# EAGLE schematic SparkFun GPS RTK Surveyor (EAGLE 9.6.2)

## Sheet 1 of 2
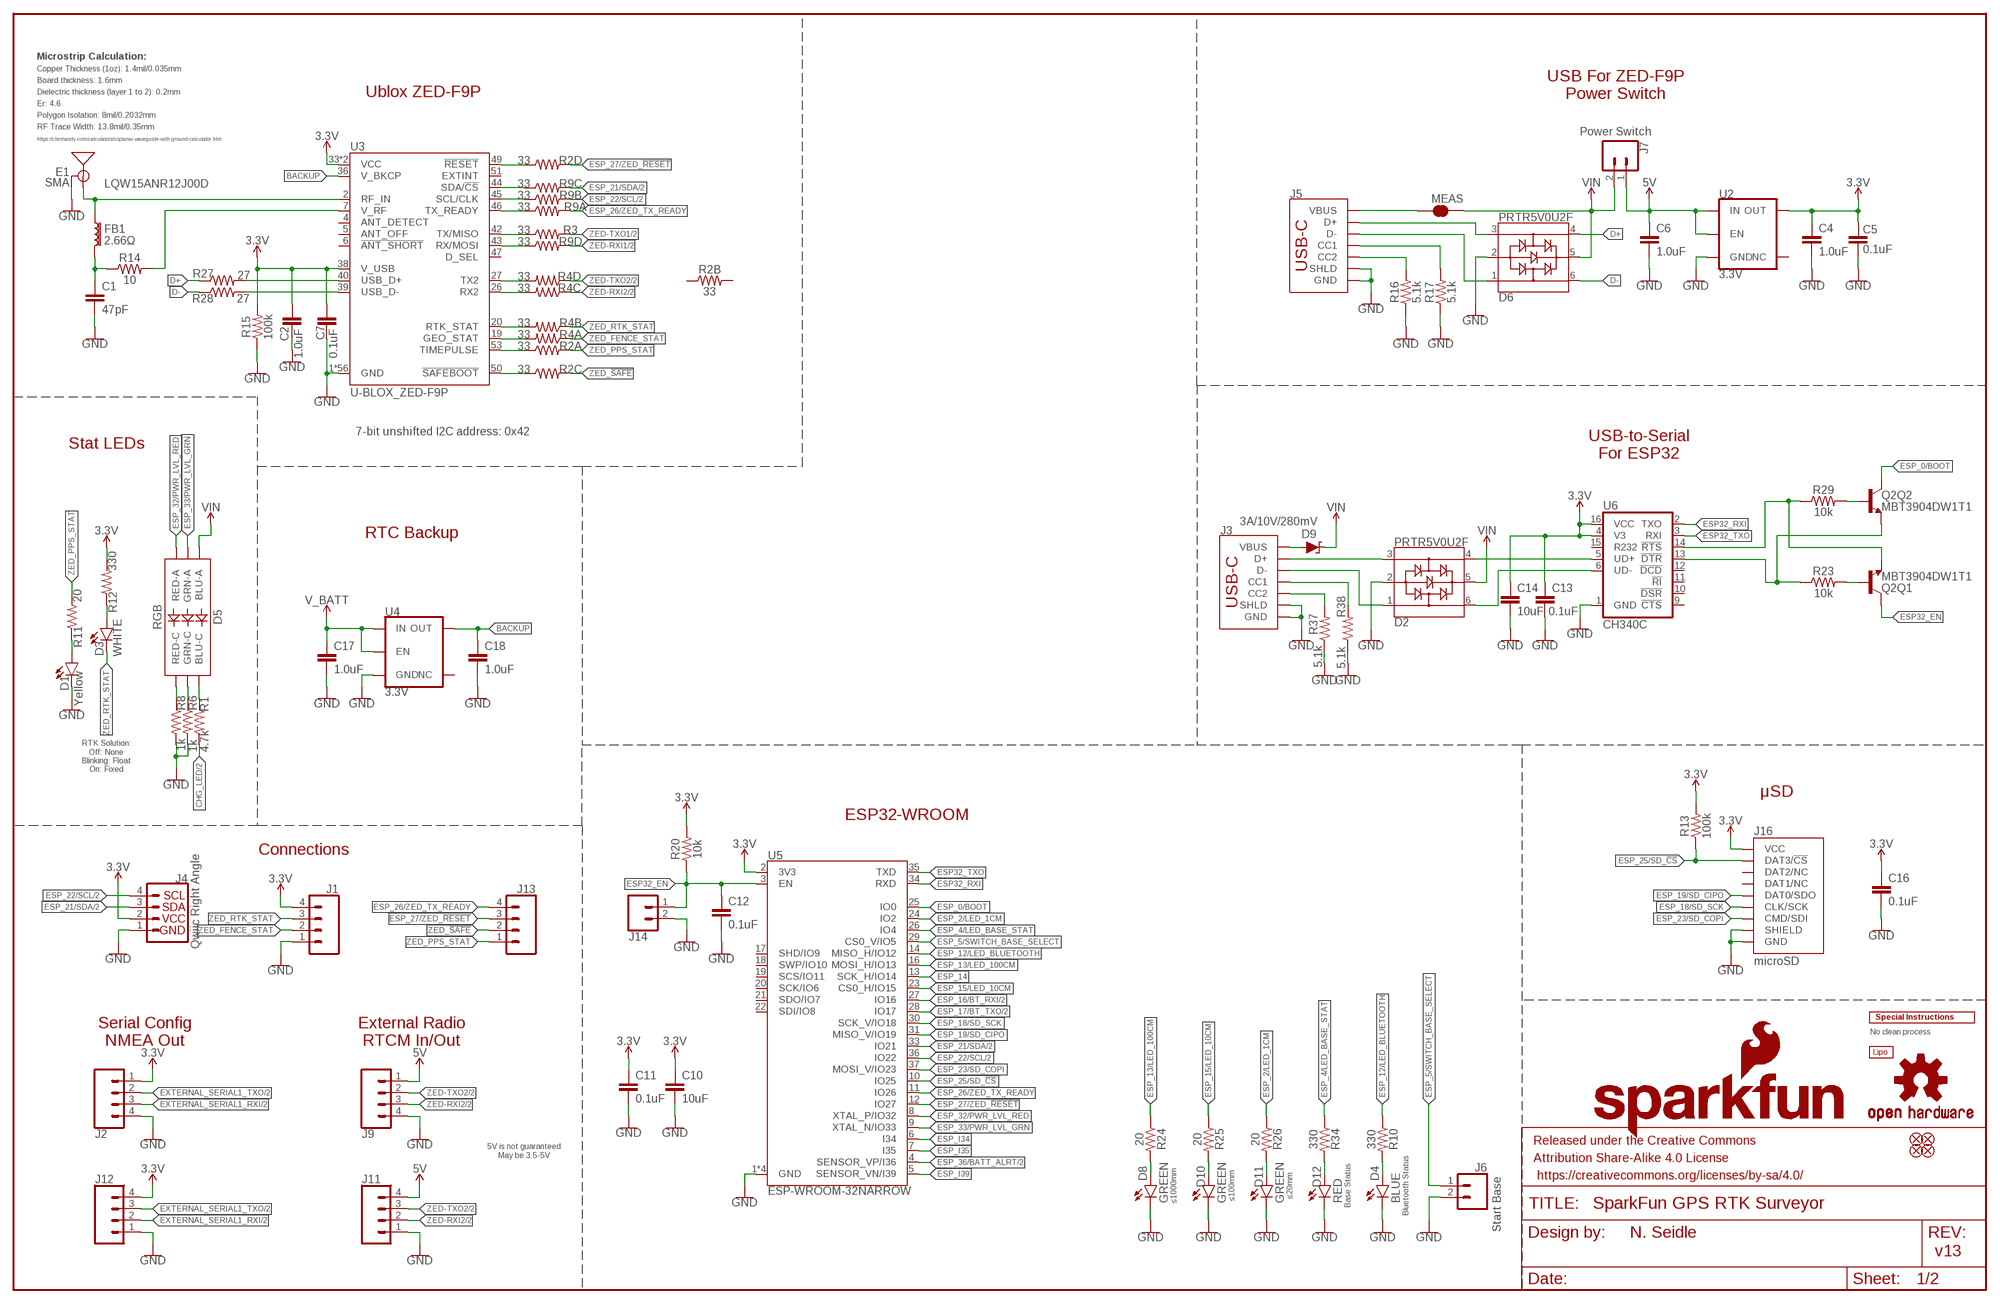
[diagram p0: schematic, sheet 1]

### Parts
BT1  LIPO-OUTLINE1100  [LIPO-1000]
C1  47pF  47PF-0402-25V-5%-X7R  [0402]
C2  1.0uF  1.0UF-0603-16V-10%-X7R  [0603]
C4  1.0uF  1.0UF-0603-16V-10%-X7R  [0603]
C5  0.1uF  0.1UF-0603-25V-5%  [0603]
C6  1.0uF  1.0UF-0603-16V-10%-X7R  [0603]
C7  0.1uF  0.1UF-0603-25V-5%  [0603]
C10  10uF  10UF-0603-6.3V-20%  [0603]
C11  0.1uF  0.1UF-0603-25V-(+80/-20%)  [0603]
C12  0.1uF  0.1UF-0603-25V-(+80/-20%)  [0603]
C13  0.1uF  0.1UF-0603-25V-(+80/-20%)  [0603]
C14  10uF  10UF-0603-6.3V-20%  [0603]
C16  0.1uF  0.1UF-0603-25V-(+80/-20%)  [0603]
C17  1.0uF  1.0UF-0603-16V-10%-X7R  [0603]
C18  1.0uF  1.0UF-0603-16V-10%-X7R  [0603]
D1  Yellow  LED-YELLOW0603  [LED-0603]
D2  PRTR5V0U2F  [SOT886]
D3  WHITE  LED-WHITE0603  [LED-0603]
D4  BLUE  LED-BLUE0603  [LED-0603]
D5  RGB  LED-RGBPLCC-6  [PLCC-6-LED]
D6  PRTR5V0U2F  [SOT886]
D8  GREEN  LED-GREEN0603  [LED-0603]
D9  3A/10V/280mV  DIODE-SCHOTTKY-BAT60A  [SOD-323]
D10  GREEN  LED-GREEN0603  [LED-0603]
D11  GREEN  LED-GREEN0603  [LED-0603]
D12  RED  LED-RED0603  [LED-0603]
E1  SMA  ANTENNA-SMA-GROUNDEDEDGE_SMA_SMD  [SMA-EDGE-SMD]
FB1  2.66Ω  FERRITE_BEAD-0402-2.66OHM-1GHZ  [0402-TIGHT]
FRAME2  FRAME-LEDGER  [CREATIVE_COMMONS]
J1  CONN_041X04_NO_SILK_NO_POP  [1X04_NO_SILK]
J2  CONN_04JST-SMD-LOCKING  [JST-4-SMD-1.25MM-LOCKING]
J3  USB Female Type C Connector  USB_C_4-LAYER_PADS  [USB-C-16P_4LAYER-PADS]
J4  Qwiic Right Angle  I2C_STANDARDQWIIC  [JST04_1MM_RA]
J5  USB Female Type C Connector  USB_C_4-LAYER_PADS  [USB-C-16P_4LAYER-PADS]
J6  Start Base  CONN_02-JST-2MM-SMT  [JST-2-SMD]
J7  Power Switch  CONN_02-JST-2MM-SMT  [JST-2-SMD]
J9  CONN_04JST-SMD-LOCKING  [JST-4-SMD-1.25MM-LOCKING]
J11  CONN_041X04_NO_SILK_NO_POP  [1X04_NO_SILK]
J12  CONN_041X04_NO_SILK_NO_POP  [1X04_NO_SILK]
J13  CONN_041X04_NO_SILK_NO_POP  [1X04_NO_SILK]
J14  CONN_021X02_NO_SILK  [1X02_NO_SILK]
J16  microSD  MICRO-SD-SDIOPUSH-PUSH  [MICRO-SD-SOCKET]
JP21  FIDUCIALUFIDUCIAL  [FIDUCIAL-MICRO]
JP61  FIDUCIALUFIDUCIAL  [FIDUCIAL-MICRO]
JP71  FIDUCIALUFIDUCIAL  [FIDUCIAL-MICRO]
JP81  FIDUCIALUFIDUCIAL  [FIDUCIAL-MICRO]
LOGO1  OSHW-LOGOMINI  [OSHW-LOGO-MINI]
LOGO2  SFE_LOGO_NAME_FLAME.1_INCH  [SFE_LOGO_NAME_FLAME_.1]
MEAS  JUMPER-COMBO_2_NC_TRACE  [COMBO-JUMPER_2_NC_TRACE]
Q2  MBT3904DW1T1  TRANS_NPN_DUAL-MBT3904DW1T1  [SC70-6]
R1  4.7k  4.7KOHM-0603-1/10W-1%  [0603]
R2  33  33OHM_RA-1206-1/16W-5%  [1206_RA]
R3  33  33OHM-0603-1/10W-1%  [0603]
R4  33  33OHM_RA-1206-1/16W-5%  [1206_RA]
R6  1k  1KOHM-0603-1/10W-1%  [0603]
R8  1k  1KOHM-0603-1/10W-1%  [0603]
R9  33  33OHM_RA-1206-1/16W-5%  [1206_RA]
R10  330  330OHM-0603-1/10W-1%  [0603]
R11  20  20OHM-0603-1/10W-1%  [0603]
R12  330  330OHM-0603-1/10W-1%  [0603]
R13  100k  100KOHM-0603-1/10W-1%  [0603]
R14  10  10OHM-0603-1/10W-1%  [0603]
R15  100k  100KOHM-0603-1/10W-1%  [0603]
R16  5.1k  5.1KOHM5.1KOHM-0603-1/10W-1%  [0603]
R17  5.1k  5.1KOHM5.1KOHM-0603-1/10W-1%  [0603]
R20  10k  10KOHM-0603-1/10W-1%  [0603]
R23  10k  10KOHM-0603-1/10W-1%  [0603]
R24  20  20OHM-0603-1/10W-1%  [0603]
R25  20  20OHM-0603-1/10W-1%  [0603]
R26  20  20OHM-0603-1/10W-1%  [0603]
R27  27  27OHM-0603-1/10W-1%  [0603]
R28  27  27OHM-0603-1/10W-1%  [0603]
R29  10k  10KOHM-0603-1/10W-1%  [0603]
R34  330  330OHM-0603-1/10W-1%  [0603]
R37  5.1k  5.1KOHM5.1KOHM-0603-1/10W-1%  [0603]
R38  5.1k  5.1KOHM5.1KOHM-0603-1/10W-1%  [0603]
U2  3.3V  V_REG_AP2112K-3.3V  [SOT23-5]
U3  U-BLOX_ZED-F9P  [ZED-F9P]
U4  3.3V  V_REG_AP2112K-3.3V  [SOT23-5]
U5  ESP-WROOM-32NARROW  [ESP-WROOM-32-NARROW]
U6  CH340C  [SO016]
U$2  SPECIAL_INSTRUCTIONS-ORDERING  [ORDERING_INSTRUCTIONS]

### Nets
3.3V [power]: C2.1 C4.1 C5.2 C7.2 C10.1 C11.1 C13.1 C14.1 C16.1 J1.4 J2.1 J4.2 J12.4 J16.VCC R12.2 R13.2 R15.2 R20.2 U2.5(OUT) U3.33(VCC) U3.34(VCC) U3.38(V_USB) U5.2(3V3) U6.4(V3) U6.16(VCC)
5V [power]: C6.1 J7.1 J9.1 J11.4 U2.1(IN) U2.3(EN)
ANT_VCC: C1.1 FB1.2 R14.1
BACKUP: C18.1 U3.36(V_BKCP) U4.5(OUT)
CC1: J5.A5(CC1) R17.2
CC2: J5.B5(CC2) R16.2
CC3: J3.B5(CC2) R37.2
CC4: J3.A5(CC1) R38.2
CHG_LED: R1.2 ; also sheet 2
D+: D6.4 R27.1
D+1: D2.4 U6.5(UD+)
D-: D6.6 R28.1
D-1: D2.6 U6.6(UD-)
ESP32_!DTR: Q2.1(Q2:E) R23.1 U6.13(!DTR)
ESP32_!RTS: Q2.4(Q1:E) R29.1 U6.14(!RTS)
ESP32_EN: C12.1 J14.1 Q2.3(Q1:C) R20.1 U5.3(EN)
ESP32_RXI: U5.34(RXD) U6.2(TXO)
ESP32_TXO: U5.35(TXD) U6.3(RXI)
ESP_0/BOOT: Q2.6(Q2:C) U5.25(IO0)
ESP_2/LED_1CM: R26.1 U5.24(IO2)
ESP_4/LED_BASE_STAT: R34.1 U5.26(IO4)
ESP_5/SWITCH_BASE_SELECT: J6.1 U5.29(CS0_V/IO5)
ESP_12/LED_BLUETOOTH: R10.1 U5.14(MISO_H/IO12)
ESP_13/LED_100CM: R24.1 U5.16(MOSI_H/IO13)
ESP_14: U5.13(SCK_H/IO14)
ESP_15/LED_10CM: R25.1 U5.23(CS0_H/IO15)
ESP_16/BT_RXI: U5.27(IO16) ; also sheet 2
ESP_17/BT_TXO: U5.28(IO17) ; also sheet 2
ESP_18/SD_SCK: J16.SCLK(CLK/SCK) U5.30(SCK_V/IO18)
ESP_19/SD_CIPO: J16.DO/DAT0(DAT0/SDO) U5.31(MISO_V/IO19)
ESP_21/SDA: J4.3 R9.P6 U5.33(IO21) ; also sheet 2
ESP_22/SCL: J4.4 R9.P7 U5.36(IO22) ; also sheet 2
ESP_23/SD_COPI: J16.DI/CMD(CMD/SDI) U5.37(MOSI_V/IO23)
ESP_25/SD_!CS!: J16.CS/DAT3(DAT3/!CS!) R13.1 U5.10(IO25)
ESP_26/ZED_TX_READY: J13.4 R9.P8 U5.11(IO26)
ESP_27/ZED_!RESET!: J13.3 R2.P5 U5.12(IO27)
ESP_32/PWR_LVL_RED: D5.AR(RED-A) U5.8(XTAL_P/IO32)
ESP_33/PWR_LVL_GRN: D5.AG(GRN-A) U5.9(XTAL_N/IO33)
ESP_36/BATT_ALRT: U5.4(SENSOR_VP/I36) ; also sheet 2
ESP_D1+: D2.3 J3.A6(D+) J3.B6(D+)
ESP_D1-: D2.1 J3.A7(D-) J3.B7(D-)
ESP_I34: U5.6(I34)
ESP_I35: U5.7(I35)
ESP_I39: U5.5(SENSOR_VN/I39)
EXTERNAL_SERIAL1_RXI: J2.3 J12.2 ; also sheet 2
EXTERNAL_SERIAL1_TXO: J2.2 J12.3 ; also sheet 2
FENCE_LV: R4.P8 U3.19(GEO_STAT)
GND: C1.2 C2.2 C4.2 C5.1 C6.2 C7.1 C10.2 C11.2 C12.2 C13.2 C14.2 C16.2 C17.2 C18.2 D1.C D2.2 D4.C D6.2 D8.C D10.C D11.C D12.C E1.GND@0(GND) E1.GND@1(GND) J1.1 J2.4 J3.GND J3.GND2(GND) J3.SHLD1(SHLD) J3.SHLD2(SHLD) J3.SHLD3(SHLD) J3.SHLD4(SHLD) J4.1 J5.GND J5.GND2(GND) J5.SHLD1(SHLD) J5.SHLD2(SHLD) J5.SHLD3(SHLD) J5.SHLD4(SHLD) J6.2 J9.4 J11.1 J12.1 J14.2 J16.CD1(SHIELD) J16.GND J16.GND1(GND) J16.GND3(GND) R6.2 R8.2 R15.1 R16.1 R17.1 R37.1 R38.1 U2.2(GND) U3.1(GND) U3.3(GND) U3.12(GND) U3.14(GND) U3.32(GND) U3.37(GND) U3.41(GND) U3.48(GND) U3.55(GND) U3.56(GND) U3.57(GND) U3.58(GND) U3.59(GND) U3.60(GND) U3.61(GND) U3.62(GND) U3.63(GND) U3.64(GND) U3.65(GND) U3.66(GND) U3.67(GND) U3.68(GND) U3.69(GND) U3.70(GND) U3.71(GND) U3.72(GND) U3.73(GND) U3.74(GND) U3.75(GND) U3.76(GND) U3.77(GND) U3.78(GND) U3.79(GND) U3.80(GND) U3.81(GND) U3.82(GND) U3.83(GND) U3.84(GND) U3.85(GND) U3.86(GND) U3.87(GND) U3.88(GND) U3.89(GND) U3.90(GND) U3.91(GND) U3.92(GND) U3.93(GND) U3.94(GND) U3.95(GND) U3.96(GND) U3.97(GND) U3.98(GND) U3.99(GND) U3.100(GND) U3.101(GND) U3.102(GND) U4.2(GND) U5.1(GND) U5.15(GND) U5.38(GND) U5.GND U6.1(GND) ; also sheet 2
GPS_ANT1 [RF]: E1.SIG(SIGNAL) FB1.1 U3.2(RF_IN)
N$1: D3.A R12.1
N$2: D1.A R11.1
N$3: D4.A R10.2
N$4 [power]: J5.VBUS1(VBUS) J5.VBUS2(VBUS) MEAS.1 MEAS.3
N$10: D5.CG(GRN-C) R6.1
N$11: R27.2 U3.40(USB_D+)
N$12: R28.2 U3.39(USB_D-)
N$13: R14.2 U3.7(V_RF)
N$14: D5.CR(RED-C) R8.1
N$16: R2.P4 U3.49(!RESET!)
N$17: D5.CB(BLU-C) R1.1
N$18: R2.P3 U3.50(!SAFEBOOT!)
N$22: R9.P1 U3.46(TX_READY)
N$24: Q2.5(Q1:B) R23.2
N$25: Q2.2(Q2:B) R29.2
N$26: D8.A R24.2
N$27: D10.A R25.2
N$29: D11.A R26.2
N$30: D12.A R34.2
N$32 [power]: D9.A J3.VBUS1(VBUS) J3.VBUS2(VBUS)
PPS: R2.P1 U3.53(TIMEPULSE)
RTK_LV: R4.P7 U3.20(RTK_STAT)
RX2_LV: R4.P6 U3.26(RX2)
RXLV: R9.P4 U3.43(RX/MOSI)
SCL_LV: R9.P2 U3.45(SCL/CLK)
SDA_LV: R9.P3 U3.44(SDA/!CS!)
TX2_LV: R4.P5 U3.27(TX2)
TXLV: R3.1 U3.42(TX/MISO)
UNP_D+: D6.3 J5.A6(D+) J5.B6(D+)
UNP_D-: D6.1 J5.A7(D-) J5.B7(D-)
V_BATT [power]: C17.1 U4.1(IN) U4.3(EN) ; also sheet 2
VIN [power]: D2.5 D5.AB(BLU-A) D6.5 D9.C J7.2 MEAS.2 MEAS.4 ; also sheet 2
ZED-RXI1: R9.P5 ; also sheet 2
ZED-RXI2: J9.3 J11.2 R4.P3 ; also sheet 2
ZED-TXO1: R3.2 ; also sheet 2
ZED-TXO2: J9.2 J11.3 R4.P4 ; also sheet 2
ZED_!SAFE!: J13.2 R2.P6
ZED_FENCE_STAT: J1.2 R4.P1
ZED_PPS_STAT: J13.1 R2.P8 R11.2
ZED_RTK_STAT: D3.C J1.3 R4.P2
Unconnected: J16.DAT1(DAT1/NC) J16.DAT2(DAT2/NC) R2.P2 R2.P7 U2.4(NC) U3.4(ANT_DETECT) U3.5(ANT_OFF) U3.6(!ANT_SHORT!) U3.47(D_SEL) U3.51(EXTINT) U4.4(NC) U5.17(SHD/IO9) U5.18(SWP/IO10) U5.19(SCS/IO11) U5.20(SCK/IO6) U5.21(SDO/IO7) U5.22(SDI/IO8) U6.9(!CTS) U6.10(!DSR) U6.11(!RI) U6.12(!DCD) U6.15(R232)

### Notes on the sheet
- Microstrip Calculation:
- Copper Thickness (1oz): 1.4mil/0.035mm
- Board thickness: 1.6mm
- USB For ZED-F9P
  Power Switch
- Ublox ZED-F9P
- Dielectric thickness (layer 1 to 2): 0.2mm
- Er: 4.6
- Polygon Isolation: 8mil/0.2032mm
- RF Trace Width: 13.8mil/0.35mm
- https://chemandy.com/calculators/coplanar-waveguide-with-ground-calculator.htm
- LQW15ANR12J00D
- 7-bit unshifted I2C address: 0x42
- Stat LEDs
- USB-to-Serial
  For ESP32
- RTC Backup
- RTK Solution:
  Off: None
  Blinking: Float
  On: Fixed
- μSD
- ESP32-WROOM
- Connections
- Serial Config
  NMEA Out
- External Radio
  RTCM In/Out
- No clean process
- 5V is not guaranteed
  May be 3.5-5V
- ≤1000mm | ≤100mm | ≤20mm | Base Status | Bluetooth Status
- N. Seidle
- v13

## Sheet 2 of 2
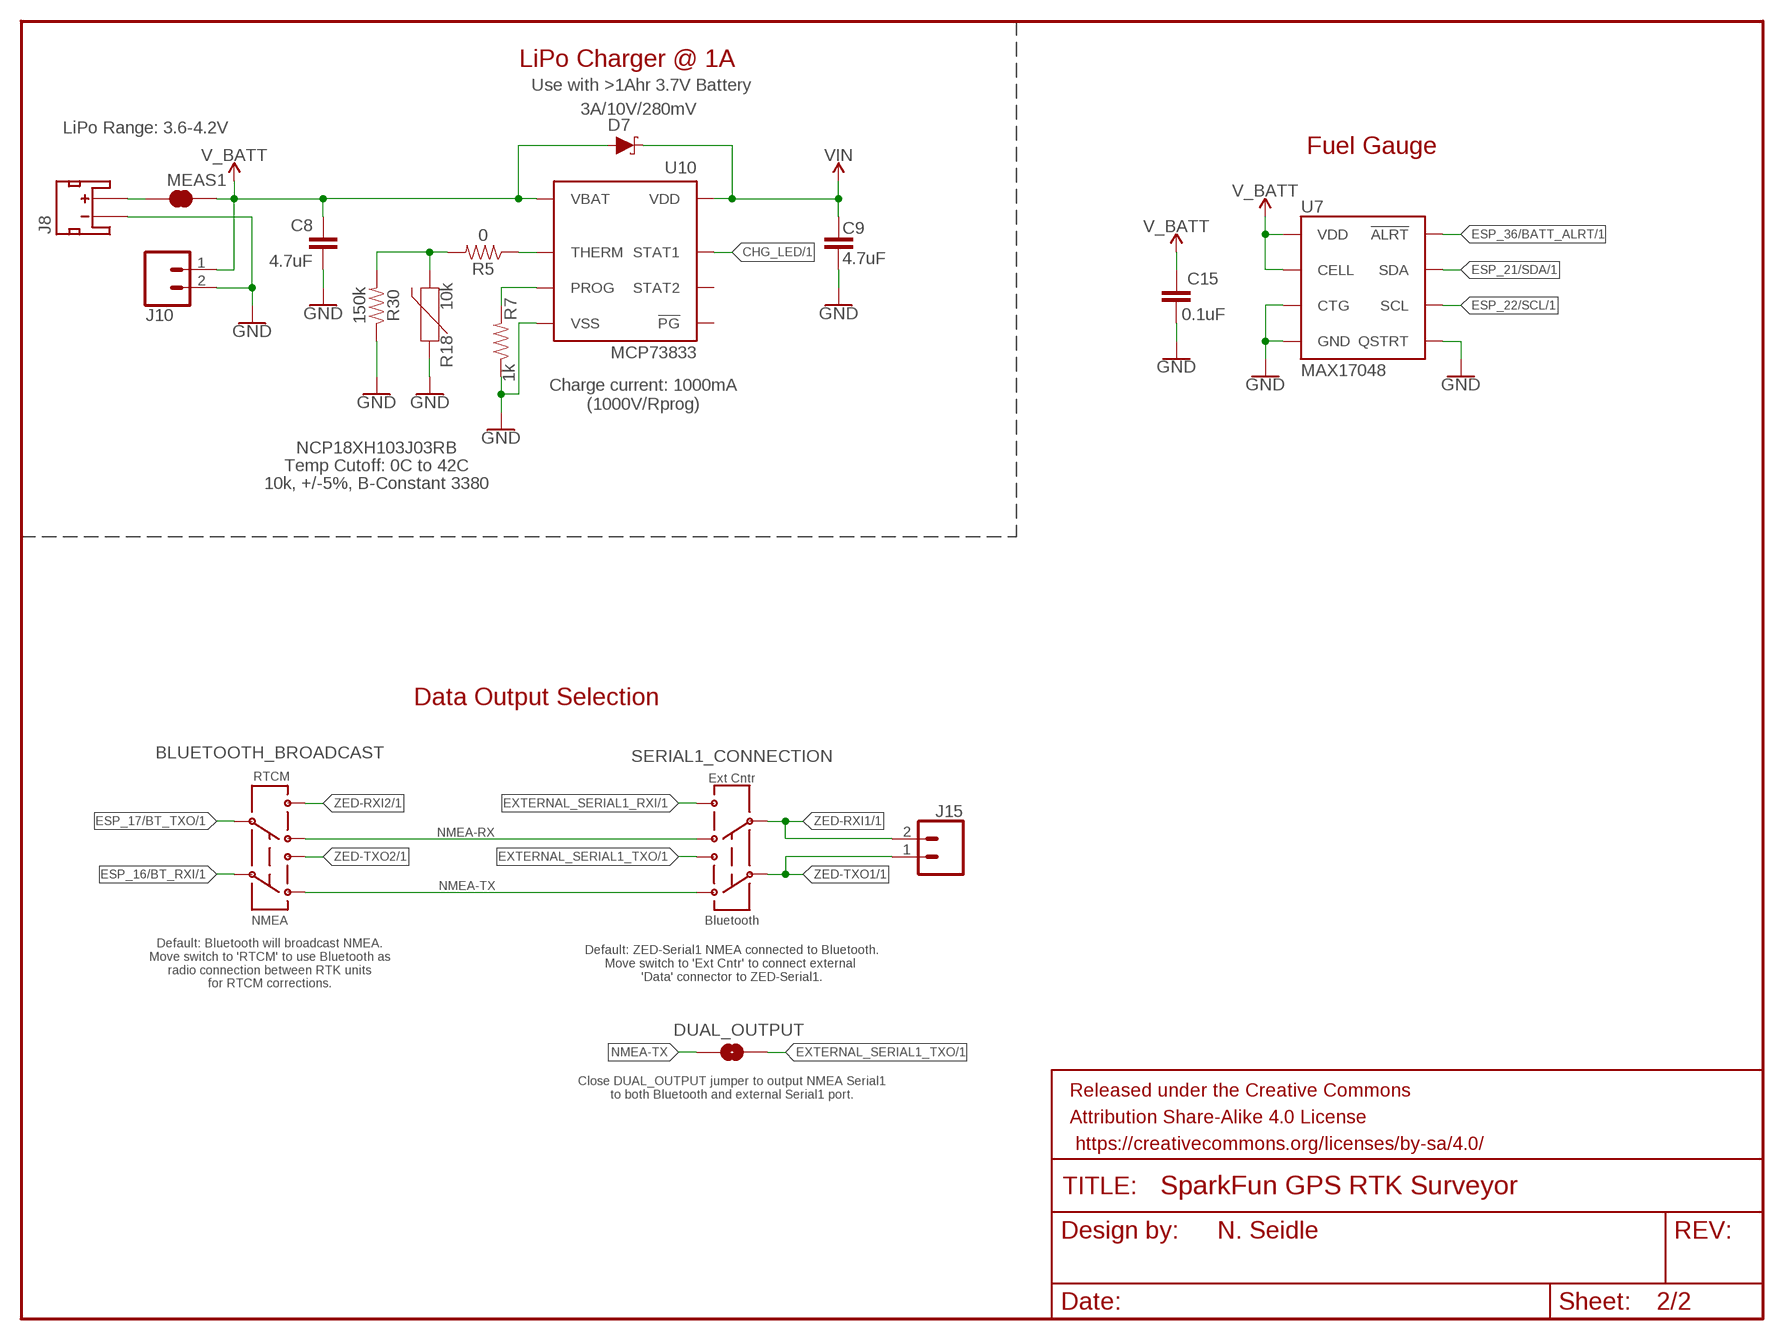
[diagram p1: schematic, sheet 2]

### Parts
BLUETOOTH_BROADCAST  SWITCH-DPDT-SMD-AYZ0202  [SWITCH_DPDT_SMD_AYZ0202]
C8  4.7uF  4.7UF-0603-35V-(20%)  [0603]
C9  4.7uF  4.7UF-0603-35V-(20%)  [0603]
C15  0.1uF  0.1UF-0603-25V-(+80/-20%)  [0603]
D7  3A/10V/280mV  DIODE-SCHOTTKY-BAT60A  [SOD-323]
DUAL_OUTPUT  JUMPER-SMT_2_NO_SILK  [SMT-JUMPER_2_NO_SILK]
FRAME1  FRAME-LETTERNO_PACKAGE  [DUMMY]
J8  JST_2MM_MALE  [JST-2-SMD]
J10  CONN_021X02_NO_SILK  [1X02_NO_SILK]
J15  CONN_021X02_NO_SILK  [1X02_NO_SILK]
MEAS1  JUMPER-COMBO_2_NC_TRACE  [COMBO-JUMPER_2_NC_TRACE]
R5  0  0OHM-0603-1/10W  [0603]
R7  1k  1KOHM-0603-1/10W-1%  [0603]
R18  10k  NTC-THERMISTOR-0603  [0603]
R30  150k  150KOHM-0603-1/10W-1%  [0603]
SERIAL1_CONNECTION  SWITCH-DPDT-SMD-AYZ0202  [SWITCH_DPDT_SMD_AYZ0202]
U7  MAX17048  MAX17048DFN8  [DFN-8]
U10  MCP73833  [DFN-10]

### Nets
CHG_LED: U10.3(STAT1) ; also sheet 1
CHG_THERM1: R5.2 R18.2 R30.2
ESP_16/BT_RXI: BLUETOOTH_BROADCAST.2 ; also sheet 1
ESP_17/BT_TXO: BLUETOOTH_BROADCAST.5 ; also sheet 1
ESP_21/SDA: U7.8(SDA) ; also sheet 1
ESP_22/SCL: U7.7(SCL) ; also sheet 1
ESP_36/BATT_ALRT: U7.5(!ALRT) ; also sheet 1
EXTERNAL_SERIAL1_RXI: SERIAL1_CONNECTION.4 ; also sheet 1
EXTERNAL_SERIAL1_TXO: DUAL_OUTPUT.2 SERIAL1_CONNECTION.1 ; also sheet 1
GND: C8.2 C9.2 C15.2 J8.1(-) J10.2 R7.1 R18.1 R30.1 U7.1(CTG) U7.4(GND) U7.6(QSTRT) U7.9(GND) U10.5(VSS) U10.11(VSS) ; also sheet 1
LIPO_RAW: J8.2(+) MEAS1.1 MEAS1.3
N$5: R5.1 U10.8(THERM)
NMEA-RX: BLUETOOTH_BROADCAST.6 SERIAL1_CONNECTION.6
NMEA-TX: BLUETOOTH_BROADCAST.3 DUAL_OUTPUT.1 SERIAL1_CONNECTION.3
PROG1: R7.2 U10.6(PROG)
V_BATT [power]: C8.1 C15.1 D7.A J10.1 MEAS1.2 MEAS1.4 U7.2(CELL) U7.3(VDD) U10.9(VBAT) U10.10(VBAT) ; also sheet 1
VIN [power]: C9.1 D7.C U10.1(VDD) U10.2(VDD) ; also sheet 1
ZED-RXI1: J15.2 SERIAL1_CONNECTION.5 ; also sheet 1
ZED-RXI2: BLUETOOTH_BROADCAST.4 ; also sheet 1
ZED-TXO1: J15.1 SERIAL1_CONNECTION.2 ; also sheet 1
ZED-TXO2: BLUETOOTH_BROADCAST.1 ; also sheet 1
Unconnected: J8.NC1(PAD1) J8.NC2(PAD2) U10.4(STAT2) U10.7(!PG)

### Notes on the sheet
- LiPo Charger @ 1A
- Use with >1Ahr 3.7V Battery
- LiPo Range: 3.6-4.2V
- Fuel Gauge
- Charge current: 1000mA
  (1000V/Rprog)
- NCP18XH103J03RB
- Temp Cutoff: 0C to 42C
- 10k, +/-5%, B-Constant 3380
- Data Output Selection
- RTCM | Ext Cntr
- NMEA | Bluetooth
- Default: Bluetooth will broadcast NMEA.
  Move switch to 'RTCM' to use Bluetooth as
  radio connection between RTK units
  for RTCM corrections.
- Default: ZED-Serial1 NMEA connected to Bluetooth.
  Move switch to 'Ext Cntr' to connect external 
  'Data' connector to ZED-Serial1.
- Close DUAL_OUTPUT jumper to output NMEA Serial1
  to both Bluetooth and external Serial1 port.
- N. Seidle

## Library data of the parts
BLUETOOTH_BROADCAST SERIAL1_CONNECTION = SparkFun-Switches:SWITCH-DPDT: Double-Pole, Double-Throw (DPDT) Switch Double-pole, double-throw switches. Variant Overview PTH-GPI-152-3013 Used on SparkFun Geiger Counter SMD-AY0202 Surface Mount DPDT Switch (COM-00597) Used on e.g. LilyPad Arduino USB - ATmega32U4 Board; PROD_ID: SWCH-08179; SF_SKU: COM-00597
BT1 = SparkFun-Batteries:LIPO-OUTLINE: LiPo Battery Outlines; PROD_ID: BATT-13243; SF_SKU: PRT-13813
C1 = SparkFun-Capacitors:47PF: 47pF ceramic capacitors; PROD_ID: CAP-15063
C2 C4 C6 C17 C18 = SparkFun-Capacitors:1.0UF: 1µF ceramic capacitors; PROD_ID: CAP-13930
C5 C7 = SparkFun-Capacitors:0.1UF: 0.1µF ceramic capacitors; PROD_ID: CAP-08604
C8 C9 = SparkFun-Capacitors:4.7UF: 4.7µF ceramic capacitors; PROD_ID: CAP-14106
C10 C14 = SparkFun-Capacitors:10UF: 10.0µF ceramic capacitors; PROD_ID: CAP-11015
C11-C13 C15 C16 = SparkFun-Capacitors:0.1UF: 0.1µF ceramic capacitors; PROD_ID: CAP-00810
D1 = SparkFun-LED:LED-YELLOW: Yellow SMD LED; PROD_ID: DIO-09003
D2 D6 = SparkFun-IC-Power:PRTR5V0U2: A small ESD protection device. Most commonly used on USB D+/D- signals to protect large, expensive, or especially sensitive USB enabled devices.; PROD_ID: DIO-14084
D3 = SparkFun-LED:LED-WHITE: White SMD LED; PROD_ID: DIO-09004
D4 = SparkFun-LED:LED-BLUE: Blue SMD LED; PROD_ID: DIO-08575
D5 = SparkFun-LED:LED-RGB: LED-RGB 6 pin RGB LED (no common connector) Packages: PLCC-6 LED-TRICOLOR-5050 - No built-in IC SparkFun Products: Digital Sandbox LED- SMD RGB; PROD_ID: DIO-12113
D7 D9 = SparkFun-DiscreteSemi:DIODE-SCHOTTKY: Schottky diode; PROD_ID: DIO-14072
D8 D10 D11 = SparkFun-LED:LED-GREEN: Green SMD LED; PROD_ID: DIO-00821
D12 = SparkFun-LED:LED-RED: Red SMD LED; PROD_ID: DIO-00819
DUAL_OUTPUT = SparkFun-Jumpers:JUMPER-SMT_2_NO: Normally open jumper
E1 = SparkFun-RF:ANTENNA-SMA-GROUNDED: SMA Antenna Connector w/ Ground; PROD_ID: CONN-15100
FB1 = SparkFun-Coils:FERRITE_BEAD: Ferrite Bead (blocks, cores, rings, chokes, etc.); PROD_ID: NDUC-15072
FRAME1 = SparkFun-Aesthetics:FRAME-LETTER: Schematic Frame - Letter; DESIGNER: Nobody; VERSION: v01
FRAME2 = SparkFun-Aesthetics:FRAME-LEDGER: Schematic Frame - Ledger
J1 J11-J13 = SparkFun-Connectors:CONN_04: Multi connection point. Often used as Generic Header-pin footprint for 0.1 inch spaced/style header connections On any of the 0.1 inch spaced packages, you can populate with these: Break Away Headers - Straight (PRT-00116) Break Away Male Headers - Right Angle (PRT-00553) Female Headers (PRT-00115)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
J2 J9 = SparkFun-Connectors:CONN_04: Multi connection point. Often used as Generic Header-pin footprint for 0.1 inch spaced/style header connections On any of the 0.1 inch spaced packages, you can populate with these: Break Away Headers - Straight (PRT-00116) Break Away Male Headers - Right Angle (PRT-00553) Female Headers (PRT-00115)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; PROD_ID: CONN-15303
J3 J5 = SparkFun-Connectors:USB_C: USB Type C 16Pin Connector Super Speed pins not available on the 16-pin purely SMD connector so this part is best for USB 2.0 implementations. D1 and D2 are tied together enabling D+/- no matter which way the cable is plugged into the connector. The two channel configuration pins (CC1/2) are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; PROD_ID: CONN-14122
J4 = SparkFun-Connectors:I2C_STANDARD: SparkFun I2C Standard Pinout Header SparkFun has standardized on a pinout for all I2C based sensor breakouts. This pinout allows I2C boards to be plugged directly into the headers on Arduino Uno compatible boards, and to be daisy chained easily. Example SparkFun Products: SparkFun Atmospheric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; PROD_ID: CONN-13694
J6 J7 = SparkFun-Connectors:CONN_02: Multi connection point. Often used as Generic Header-pin footprint for 0.1 inch spaced/style header connections; PROD_ID: CONN-11443
J8 = SparkFun-Connectors:JST_2MM_MALE: JST 2MM MALE RA CONNECTOR Two pin, compact surface mount connector. Commonly used as a battery input connection point. We really like the solid locking feeling and high current rating on these small connectors. We use these all the time as battery connectors. Mates to single-cell LiPo batteries.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; PROD_ID: CONN-11443; SF_ID: PRT-08612
J10 J14 J15 = SparkFun-Connectors:CONN_02: Multi connection point. Often used as Generic Header-pin footprint for 0.1 inch spaced/style header connections
J16 = SparkFun-Connectors:MICRO-SD-SDIO: microSD Socket for Transflash Push-push type µSD socket. tDoc lines correctly indicate media card edge positions when inserting (unlocked, locked, depressed). NOTE: CD1 and CD2 are connected internally, and the default detect state of the socket is detect pin to ground. SparkFun Products: WAV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; PROD_ID: CONN-07820
JP21 JP61 JP71 JP81 = SparkFun-Aesthetics:FIDUCIAL: Fiducial Alignment Points
LOGO1 = SparkFun-Aesthetics:OSHW-LOGO: Open-Source Hardware (OSHW) Logo
LOGO2 = SparkFun-Aesthetics:SFE_LOGO_NAME_FLAME: SparkFun Font Logo w/ Flame
MEAS MEAS1 = SparkFun-Jumpers:JUMPER-COMBO_2_NC_TRACE
Q2 = SparkFun-DiscreteSemi:TRANS_NPN_DUAL: Dual NPN Transistors in Single Package The MBT3904W1 puts two general purpose 3904 NPN transistors in a single package. Datasheet SparkFun Products: SparkFun ESP32 Thing; PROD_ID: TRANS-13337
R1 = SparkFun-Resistors:4.7KOHM: 4.7kΩ resistor; PROD_ID: RES-07857
R2 R4 R9 = SparkFun-Resistors:33OHM_RA: EXB-38V330JV Four Resistory Array - AEC-Q200 Certified; PROD_ID: RES-15081
R3 = SparkFun-Resistors:33OHM: 33Ω resistor; PROD_ID: RES-08270
R5 = SparkFun-Resistors:0OHM: 0Ω resistor; PROD_ID: RES-08609
R6-R8 = SparkFun-Resistors:1KOHM: 1kΩ resistor; PROD_ID: RES-07856
R10 R12 R34 = SparkFun-Resistors:330OHM: 330Ω resistor; PROD_ID: RES-00818
R11 R24-R26 = SparkFun-Resistors:20OHM: RES-07862; PROD_ID: RES-07862
R13 R15 = SparkFun-Resistors:100KOHM: 100kΩ resistor; PROD_ID: RES-07828
R14 = SparkFun-Resistors:10OHM: 10Ω resistor; PROD_ID: RES-12581
R16 R17 R37 R38 = SparkFun-Resistors:5.1KOHM; PROD_ID: RES-12083
R18 = SparkFun-Resistors:NTC-THERMISTOR: NTC Thermistor; PROD_ID: RES-13608
R20 R23 R29 = SparkFun-Resistors:10KOHM: 10kΩ resistor; PROD_ID: RES-00824
R27 R28 = SparkFun-Resistors:27OHM: 27Ω resistor; PROD_ID: RES-09334
R30 = SparkFun-Resistors:150KOHM: 150kΩ resistor; PROD_ID: RES-09117
U2 U4 = SparkFun-IC-Power:V_REG_AP2112: AP2112 - 600mA CMOS LDO Regulator w/ Enable The AP2112 is CMOS process low dropout linear regulator with enable function, the regulator delivers a guaranteed 600mA (min.) continuous load current. Features Output Voltage Accuracy: ±1.5% Output Current: 600mA (Min.) Foldback Short Current Protection: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; PROD_ID: VREG-12457
U3 = SparkFun-GPS:U-BLOX_ZED-F9P; PROD_ID: IC-14209
U5 = SparkFun-RF:ESP-WROOM-32; PROD_ID: IC-13849
U6 = SparkFun-IC-Comms:CH340C; PROD_ID: IC-14038
U7 = SparkFun-IC-Power:MAX17048: Micropower 1-Cell Li+ ModelGauge SparkFun Products Qduino Mini (DEV-13614); PROD_ID: IC-12551
U10 = SparkFun-IC-Power:MCP73833; PROD_ID: IC-14369
U$2 = SparkFun-Aesthetics:SPECIAL_INSTRUCTIONS: Special Ordering/Production Instructions Alert

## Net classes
1 power: width 0.305 mm
2 3.3V: width 0.559 mm
3 RF: width 0.35 mm, clearance 0.203 mm

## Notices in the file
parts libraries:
SparkFun-Resistors: Licensing: Creative Commons ShareAlike 4.0 International - https://creativecommons.org/licenses/by-sa/4.0
SparkFun-Aesthetics: Released under the Creative Commons Attribution Share-Alike 4.0 License
SparkFun-Aesthetics: https://creativecommons.org/licenses/by-sa/4.0
